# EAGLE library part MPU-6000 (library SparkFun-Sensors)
Invensense MPU-6000 6-Axis Gryoscope/Accelerometer 3-axis gyroscope, 3-axis accelerometer in a 4x4 package. The MPU-6000 is the world’s first 6-axis I²C MotionTracking device designed for the low power, low cost, and high performance requirements of smartphones, tablets and wearable sensors. Datasheet SparkFun Products MPU-6000 - Motion Processing Unit (SEN-11234) SparkFun UDB5 - PIC UAV Development Board (GPS-11703)
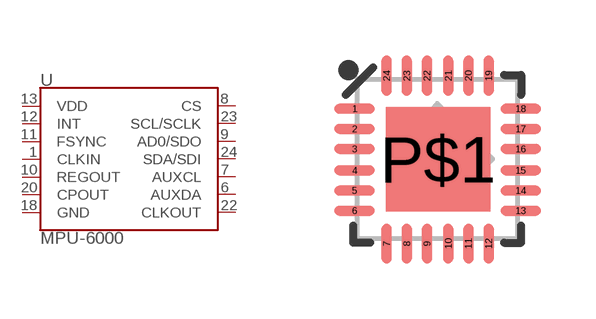
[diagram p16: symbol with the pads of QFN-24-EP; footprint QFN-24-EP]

Designator prefix U

## MPU-6000 (PROD_ID: IC-11089; SF_ID: SEN-11234)  [QFN-24-EP]
1  CLKIN
6  AUXDA
7  AUXCL
8  CS
9  AD0/SDO
10  REGOUT
11  FSYNC
12  INT
13  VDD
18  GND
20  CPOUT
22  CLKOUT
23  SCL/SCLK
24  SDA/SDI

## Footprint QFN-24-EP (pad centres in mm)
24-Pin QFN w/ Center Pad (4 x 4 mm) Datasheet Specifications: Pin Count: 24 Area: 4.0 x 4.0 x 0.90 mm Pitch: 0.5 mm Devices Using: MPU-6000
smd 1.016 x 0.254: 1 -2.066,1.257; 2 -2.066,0.75; 3 -2.066,0.247; 4 -2.066,-0.287; 5 -2.066,-0.792; 6 -2.066,-1.297; 13 2.086,-1.297; 14 2.086,-0.792; 15 2.086,-0.287; 16 2.086,0.247; 17 2.086,0.75; 18 2.086,1.257
smd 0.254 x 1.016: 7 -1.267,-2.122; 8 -0.762,-2.122; 9 -0.258,-2.122; 10 0.278,-2.122; 11 0.78,-2.122; 12 1.287,-2.122; 19 1.287,2.082; 20 0.78,2.082; 21 0.278,2.082; 22 -0.258,2.082; 23 -0.762,2.082; 24 -1.267,2.082
smd 2.616 x 2.616: P$1 0.02,-0.01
